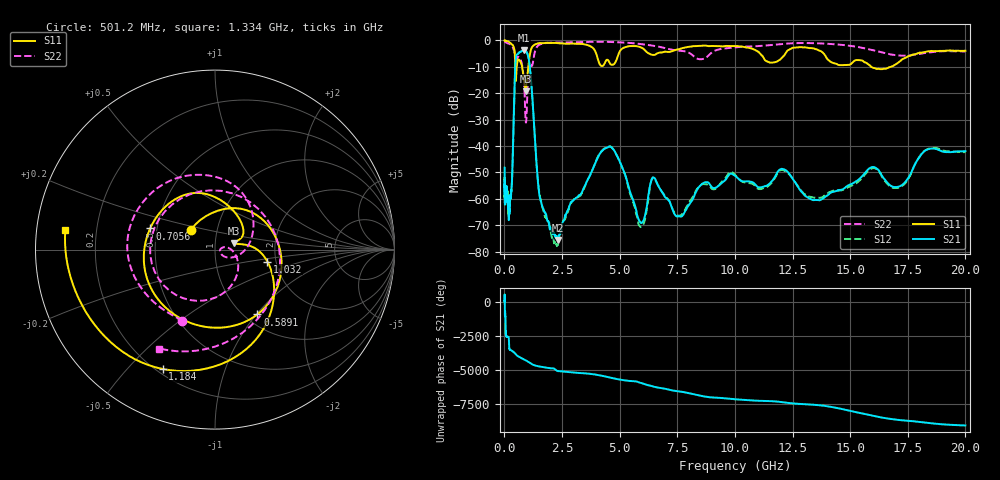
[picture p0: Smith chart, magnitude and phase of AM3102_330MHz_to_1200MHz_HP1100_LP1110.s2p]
! Date/Time: Tue, Sep 11, 2018 5:21 PM
! Network Analyzer: Agilent Technologies E8362B Rev: A.07.50.63
! Sweep from 0.010 to 20.000 GHz, 1601 Points, Sweep Type: LOG
! Power Supply: 4.949 V, 0.001 A
# Hz S DB R 50
!freq MagS11 AngS11 MagS21 AngS21 MagS12 AngS12 MagS22 AngS22
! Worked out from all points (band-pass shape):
!   1601 points, 10 MHz to 20 GHz, reference 50 ohm
!   highest |S21| = -3.63 dB at 849.3 MHz (marker M1); lowest = -75.5 dB at 2.314 GHz (marker M2)
!   |S21| within 3 dB of the highest: 497.6 MHz to 1.047 GHz (549 MHz wide, 71.1 % of centre)
!   lowest |S11| = -19.2 dB at 925.1 MHz (marker M3), VSWR 1.25, Z = 61.4 + j4.36 ohm
!   |S11| at or under -10 dB: 471 MHz to 535.2 MHz (64.24 MHz wide, 12.8 % of centre); 769.1 MHz to 1.038 GHz (268.4 MHz wide, 29.7 % of centre); 15.92 GHz to 16.76 GHz (842.8 MHz wide, 5.16 % of centre)
!   |S22| runs from -31.1 to -0.2 dB; largest |S21 - S12| = 0.0094
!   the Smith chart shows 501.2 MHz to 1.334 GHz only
!   S11 on the Smith chart (normalised r, x): 501.2 MHz: 0.75, +0.17; 589.1 MHz: 1.14, -1.01; 705.6 MHz: 0.46, +0.13; 1.032 GHz: 1.80, -0.27; 1.184 GHz: 0.22, -0.63; 1.334 GHz: 0.09, +0.06
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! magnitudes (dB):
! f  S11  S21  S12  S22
! 10 MHz  0.0  -48.2  -52.9  -0.2
! 35.55 MHz  -0.1  -59.3  -58.4  -0.5
! 126.4 MHz  -0.3  -58.3  -58.4  -1.0
! 192 MHz  -0.5  -68.0  -66.6  -1.2
! 316.2 MHz  -1.5  -54.9  -56.1  -2.0
! 447.2 MHz  -4.6  -15.6  -15.7  -4.7
! 501.2 MHz  -15.2  -6.4  -6.4  -7.2
! 589.1 MHz  -7.3  -5.0  -5.1  -6.2
! 705.6 MHz  -8.4  -4.2  -4.3  -7.4
! 849.3 MHz  -14.6  -3.6  -3.7  -15.3
! 925.1 MHz  -19.2  -3.9  -3.9  -30.7
! 1.032 GHz  -10.5  -6.1  -6.0  -14.0
! 1.184 GHz  -2.8  -18.0  -18.0  -9.7
! 1.334 GHz  -1.5  -38.5  -38.9  -4.0
! 1.59 GHz  -1.0  -61.2  -60.8  -1.3
! 2.314 GHz  -1.0  -75.5  -77.5  -0.8
! 4.436 GHz  -7.3  -40.7  -40.5  -0.5
! 5.652 GHz  -2.1  -62.2  -63.1  -1.1
! 7.625 GHz  -3.2  -66.7  -66.3  -3.9
! 12.09 GHz  -6.1  -48.7  -49.1  -1.3
! 13.61 GHz  -3.7  -60.5  -59.6  -1.1
! 20 GHz  -3.9  -41.9  -42.4  -4.2
